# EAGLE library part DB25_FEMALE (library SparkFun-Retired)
25 Pin male connector. PCB edge mount for regular PCB thicknesses. This connector will connect directly to the back of a PC parallel port or through a normal DB25 extension cable (M/F). SKU: PRT-08287
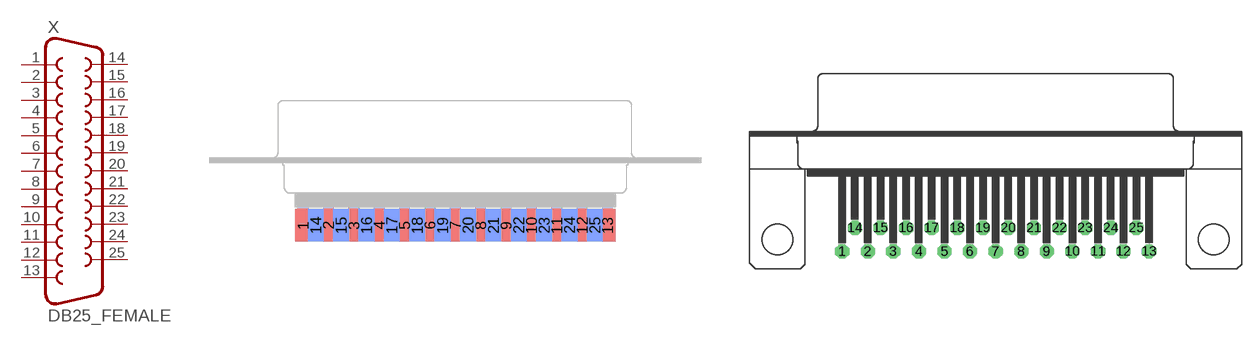
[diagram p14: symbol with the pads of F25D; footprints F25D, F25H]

Designator prefix X

## DB25_FEMALED  [F25D]
1  1  pas
2  2  pas
3  3  pas
4  4  pas
5  5  pas
6  6  pas
7  7  pas
8  8  pas
9  9  pas
10  10  pas
11  11  pas
12  12  pas
13  13  pas
14  14  pas
15  15  pas
16  16  pas
17  17  pas
18  18  pas
19  19  pas
20  20  pas
21  21  pas
22  22  pas
23  23  pas
24  24  pas
25  25  pas

## DB25_FEMALEH  [F25H]
Pads as for F25D

## DB25_FEMALEHP  [F25HP]
Pads as for F25D

## DB25_FEMALEV  [F25V]
Pads as for F25D

## DB25_FEMALEVP  [F25VP]
Pads as for F25D

## DB25_FEMALEVB  [F25VB]
Pads as for F25D

## Footprint F25D (pad centres in mm)
SUB-D
smd 1.7 x 3.5: 1 -16.459,-6.045; 2 -13.716,-6.045; 3 -10.973,-6.045; 4 -8.23,-6.045; 5 -5.486,-6.045; 6 -2.743,-6.045; 7 0,-6.045; 8 2.743,-6.045; 9 5.486,-6.045; 10 8.23,-6.045; 11 10.973,-6.045; 12 13.716,-6.045; 13 16.459,-6.045
smd 1.7 x 3.5 bottom: 14 -15.088,-6.045; 15 -12.344,-6.045; 16 -9.601,-6.045; 17 -6.858,-6.045; 18 -4.115,-6.045; 19 -1.372,-6.045; 20 1.372,-6.045; 21 4.115,-6.045; 22 6.858,-6.045; 23 9.601,-6.045; 24 12.344,-6.045; 25 15.088,-6.045

## Footprint F25H (pad centres in mm)
SUB-D
drill 1.016 octagon: 1 -16.561,-1.27; 2 -13.792,-1.27; 3 -11.049,-1.27; 4 -8.28,-1.27; 5 -5.512,-1.27; 6 -2.769,-1.27; 7 0,-1.27; 8 2.769,-1.27; 9 5.512,-1.27; 10 8.28,-1.27; 11 11.049,-1.27; 12 13.792,-1.27; 13 16.561,-1.27; 14 -15.189,1.27; 15 -12.421,1.27; 16 -9.652,1.27; 17 -6.909,1.27; 18 -4.14,1.27; 19 -1.372,1.27; 20 1.372,1.27; 21 4.14,1.27; 22 6.909,1.27; 23 9.652,1.27; 24 12.421,1.27; 25 15.189,1.27
hole 3.302 at -23.52,0
hole 3.302 at 23.52,0

## Footprint F25HP (pad centres in mm)
SUB-D
drill 1.016 octagon: 1 -16.561,-1.27; 2 -13.792,-1.27; 3 -11.049,-1.27; 4 -8.28,-1.27; 5 -5.512,-1.27; 6 -2.769,-1.27; 7 0,-1.27; 8 2.769,-1.27; 9 5.512,-1.27; 10 8.28,-1.27; 11 11.049,-1.27; 12 13.792,-1.27; 13 16.561,-1.27; 14 -15.189,1.27; 15 -12.421,1.27; 16 -9.652,1.27; 17 -6.909,1.27; 18 -4.14,1.27; 19 -1.372,1.27; 20 1.372,1.27; 21 4.14,1.27; 22 6.909,1.27; 23 9.652,1.27; 24 12.421,1.27; 25 15.189,1.27
drill 3.302 pad 5.08: G1 -23.52,0; G2 23.52,0

## Footprint F25V (pad centres in mm)
SUB-D
drill 1.016 octagon: 1 16.561,1.422; 2 13.792,1.422; 3 11.049,1.422; 4 8.28,1.422; 5 5.512,1.422; 6 2.769,1.422; 7 0,1.422; 8 -2.769,1.422; 9 -5.512,1.422; 10 -8.28,1.422; 11 -11.049,1.422; 12 -13.792,1.422; 13 -16.561,1.422; 14 15.189,-1.422; 15 12.421,-1.422; 16 9.652,-1.422; 17 6.909,-1.422; 18 4.14,-1.422; 19 1.372,-1.422; 20 -1.372,-1.422; 21 -4.14,-1.422; 22 -6.909,-1.422; 23 -9.652,-1.422; 24 -12.421,-1.422; 25 -15.189,-1.422
hole 3.302 at 23.52,0
hole 3.302 at -23.52,0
